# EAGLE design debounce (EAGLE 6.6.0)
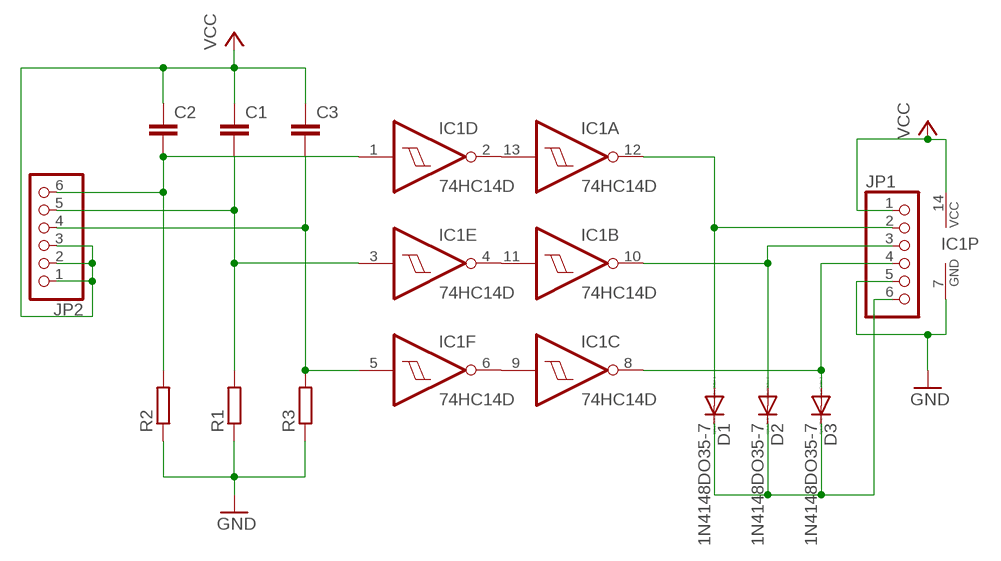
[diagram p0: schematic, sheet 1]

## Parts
C1  C-EU050-024X044  [C050-024X044]
C2  C-EU050-024X044  [C050-024X044]
C3  C-EU050-024X044  [C050-024X044]
D1  1N4148DO35-7  [DO35-7]
D2  1N4148DO35-7  [DO35-7]
D3  1N4148DO35-7  [DO35-7]
IC1  74HC14D  [SO14]
JP1  PINHD-1X6  [1X06]
JP2  PINHD-1X6  [1X06]
R1  R-EU_0207/10  [0207/10]
R2  R-EU_0207/10  [0207/10]
R3  R-EU_0207/10  [0207/10]

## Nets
GND: IC1.7(P:GND) JP1.5 R1.1 R2.1 R3.1
N$1: IC1.2(D:O) IC1.13(A:I)
N$2: IC1.4(E:O) IC1.11(B:I)
N$3: IC1.6(F:O) IC1.9(C:I)
N$4: D3.A IC1.8(C:O) JP1.4
N$5: C2.2 IC1.1(D:I) JP2.6 R2.2
N$6: C1.2 IC1.3(E:I) JP2.5 R1.2
N$7: C3.2 IC1.5(F:I) JP2.4 R3.2
N$8: D2.A IC1.10(B:O) JP1.3
N$10: D1.C D2.C D3.C JP1.6
N$11: D1.A IC1.12(A:O) JP1.2
VCC: C1.1 C2.1 C3.1 IC1.14(P:VCC) JP1.1 JP2.1 JP2.2 JP2.3

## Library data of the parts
C1-C3 = rcl:C-EU: CAPACITOR, European symbol
D1-D3 = diode:1N4148: DIODE
IC1 = 74xx-eu:74*14: Hex schmitt trigger INVERTER
JP1 JP2 = pinhead:PINHD-1X6: PIN HEADER
R1-R3 = rcl:R-EU_: RESISTOR, European symbol

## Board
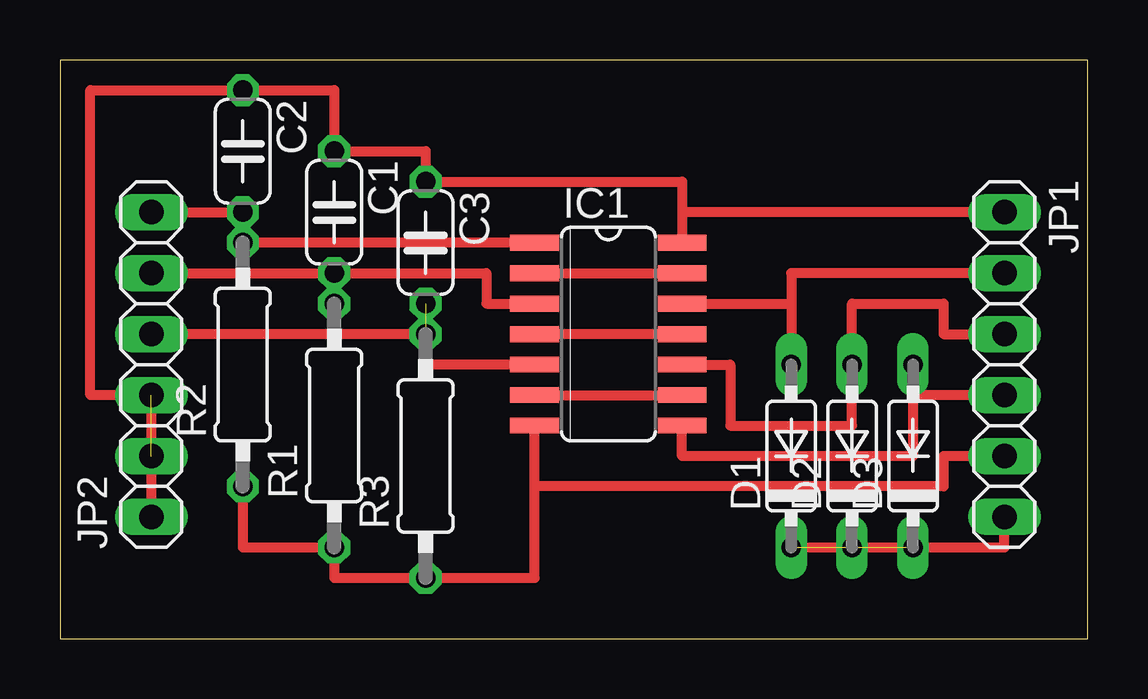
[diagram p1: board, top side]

Size 42.85 x 24.12 mm. Coordinates in mm from the lower left corner, seen from the top.
Outline: 0,0 42.85,0 42.85,24.12 0,24.12 0,0
Copper layers (1*16): Top 0.035mm / dielectric 1.5mm / Bottom 0.035mm
Design rules "default": minimum track width 10mil, minimum drill 24mil, track to track 8mil, track to pad 8mil, pad to pad 8mil, via to via 8mil, smd to smd 8mil, copper to edge 40mil, drill to drill 8mil, minimum pad ring 10mil, minimum via ring 8mil, stop-mask expansion 4mil, vias tented up to drill 0mil, thermal gap 10mil

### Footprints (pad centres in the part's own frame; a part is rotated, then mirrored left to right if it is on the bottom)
C050-024X044 = drill 0.813 octagon: 1 -2.54,0; 2 2.54,0
DO35-7 = drill 0.813 long: A 3.81,0; C -3.81,0
SO14 = smd 0.66 x 2.032: 1 -3.81,-3.073; 2 -2.54,-3.073; 3 -1.27,-3.073; 4 0,-3.073; 5 1.27,-3.073; 6 2.54,-3.073; 7 3.81,-3.073; 8 3.81,3.073; 9 2.54,3.073; 10 1.27,3.073; 11 0,3.073; 12 -1.27,3.073; 13 -2.54,3.073; 14 -3.81,3.073
1X06 = drill 1.016 long: 1 -6.35,0; 2 -3.81,0; 3 -1.27,0; 4 1.27,0; 5 3.81,0; 6 6.35,0
0207/10 = drill 0.813 octagon: 1 -5.08,0; 2 5.08,0

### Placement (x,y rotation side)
C1  11.43,17.78 270 top
C2  7.62,20.32 270 top
C3  15.24,16.51 270 top
D1  30.48,7.62 90 top
D2  33.02,7.62 90 top
D3  35.56,7.62 90 top
IC1  22.86,12.7 270 top
JP1  39.37,11.43 270 top
JP2  3.81,11.43 90 top
R1  11.43,8.89 90 top
R2  7.62,11.43 90 top
R3  15.24,7.62 90 top

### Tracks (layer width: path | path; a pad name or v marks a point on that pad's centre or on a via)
GND
  Top 0.406: R2.1 7.62,3.81 R1.1 11.43,2.54 R3.1 19.79,2.54 19.79,6.35 | 19.79,6.35 IC1.7 | JP1.5 36.83,7.62 36.83,6.35 19.79,6.35
N$1
  Top 0.406: IC1.2 IC1.13
N$2
  Top 0.406: IC1.11 IC1.4
N$3
  Top 0.406: IC1.6 IC1.9
N$4  (1 unrouted)
  Top 0.406: JP1.4 35.56,10.16 35.56,8.89 | D3.A 35.56,7.62 25.93,7.62 IC1.8
N$5
  Top 0.406: JP2.6 C2.2 R2.2 IC1.1
N$6
  Top 0.406: JP2.5 C1.2 | R1.2 C1.2 | C1.2 17.78,15.24 17.78,13.97 IC1.3 20.32,13.97
N$7  (1 unrouted)
  Top 0.406: IC1.5 15.24,11.43 R3.2 | R3.2 C3.2 | R3.2 JP2.4
N$8
  Top 0.406: IC1.10 27.94,11.43 27.94,8.89 33.02,8.89 D2.A 33.02,13.97 36.83,13.97 36.83,12.7 JP1.3
N$10  (2 unrouted)
  Top 0.406: D1.C 39.37,3.81 JP1.6
N$11
  Top 0.406: JP1.2 30.48,15.24 30.48,13.97 | 30.48,13.97 D1.A | IC1.12 30.48,13.97
VCC  (1 unrouted)
  Top 0.406: JP2.1 JP2.3 1.27,10.16 1.27,22.86 C2.1 11.43,22.86 C1.1 15.24,20.32 C3.1 25.93,19.05 IC1.14 25.93,17.78 JP1.1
